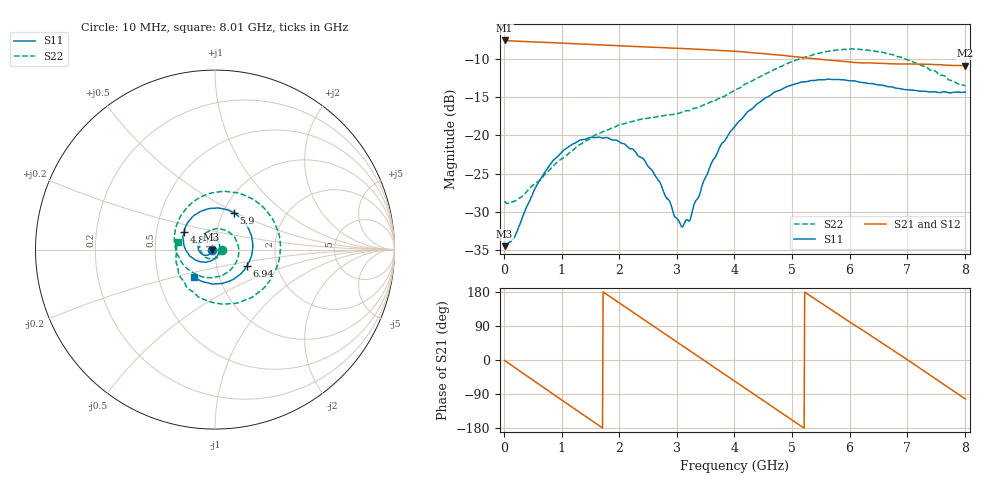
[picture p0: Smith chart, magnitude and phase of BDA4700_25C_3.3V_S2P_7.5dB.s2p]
!Agilent Technologies,E5071B,MY42404982,A.09.10
!Date: Mon Oct 20 18:06:09 2025
!Data & Calibration Information:
!Freq	S11:SOLT2(ON)	S21:SOLT2(ON)	S12:SOLT2(ON)	S22:SOLT2(ON)
# Hz S RI R 50
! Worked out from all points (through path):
!   801 points, 10 MHz to 8.01 GHz, reference 50 ohm
!   highest |S21| = -7.61 dB at 10 MHz (marker M1); lowest = -10.9 dB at 8.01 GHz (marker M2)
!   group delay of S21, straight-line fit = 285 ps
!   lowest |S11| = -34.5 dB at 10 MHz (marker M3), VSWR 1.04, Z = 48.1 - j0.0879 ohm
!   |S11| at or under -10 dB: start of sweep to end of sweep
!   |S22| runs from -28.9 to -8.7 dB; largest |S21 - S12| = 0.0047
!   S11 on the Smith chart (normalised r, x): 10 MHz: 0.96, -0.00; 4.81 GHz: 0.69, +0.14; 5.9 GHz: 1.12, +0.49; 6.94 GHz: 1.40, -0.27; 8.01 GHz: 0.76, -0.24
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1e7  -0.0189 -0.000913  0.4161 -0.00863  0.416 -0.00924  0.0372 -0.0028
3.3e8  -0.0236 -0.0184  0.3347 -0.2365  0.3347 -0.2368  0.0243 -0.0322
7.1e8  -0.048 -0.0318  0.1034 -0.3908  0.1032 -0.3911  -0.0183 -0.0525
1.02e9  -0.0755 -0.023  -0.1207 -0.3808  -0.1205 -0.381  -0.0619 -0.0345
1.35e9  -0.0936 0.00545  -0.3106 -0.2431  -0.3107 -0.2431  -0.0856 0.0221
1.64e9  -0.0896 0.0383  -0.3863 -0.0537  -0.3861 -0.054  -0.0653 0.0791
1.93e9  -0.0674 0.0644  -0.3571 0.1452  -0.357 0.1452  -0.00557 0.1135
2.32e9  -0.023 0.0704  -0.1763 0.336  -0.1761 0.3358  0.0883 0.0896
2.68e9  0.0141 0.0488  0.0611 0.3696  0.0605 0.3693  0.1328 0.000702
3.11e9  0.0248 -0.00624  0.2973 0.2178  0.2956 0.2192  0.0854 -0.1144
3.23e9  0.0192 -0.0207  0.3349 0.1498  0.3349 0.1491  0.0548 -0.135
3.54e9  -0.0115 -0.0562  0.3586 -0.0491  0.3584 -0.0501  -0.0425 -0.1562
4.01e9  -0.0959 -0.0633  0.1955 -0.2949  0.196 -0.2942  -0.1821 -0.0762
4.39e9  -0.1598 -0.00836  -0.034 -0.3427  -0.0339 -0.3432  -0.2267 0.0658
4.81e9  -0.1724 0.099  -0.2523 -0.2186  -0.2504 -0.22  -0.1553 0.2351
5.35e9  -0.0701 0.2167  -0.3081 0.0778  -0.3084 0.076  0.0944 0.32
5.9e9  0.1043 0.2052  -0.1063 0.2848  -0.1071 0.2841  0.3317 0.1493
6.28e9  0.1874 0.1147  0.0846 0.2845  0.0884 0.2822  0.3556 -0.0626
6.68e9  0.2073 -0.0149  0.2461 0.16  0.2468 0.1594  0.2354 -0.2444
6.94e9  0.1773 -0.0915  0.2899 0.0363  0.2901 0.0346  0.1089 -0.2991
7.6e9  -8.95e-05 -0.1914  0.1418 -0.2514  0.1413 -0.2516  -0.1906 -0.1561
8.01e9  -0.1182 -0.1512  -0.064 -0.2773  -0.0633 -0.2776  -0.2066 0.0424
